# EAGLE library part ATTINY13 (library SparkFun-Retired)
ATTINY13 Retired
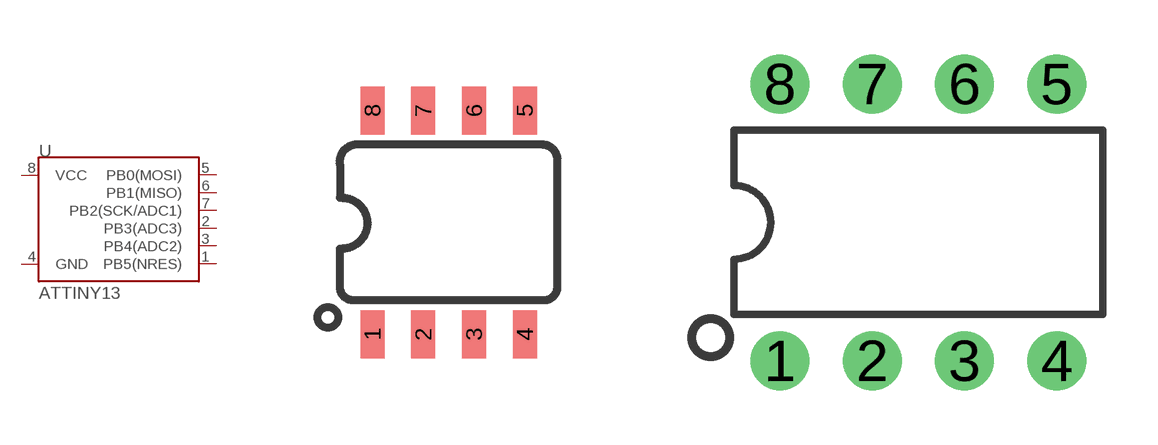
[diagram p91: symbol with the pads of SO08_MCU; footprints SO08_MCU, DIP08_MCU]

Designator prefix -

## ATTINY13SOIC  [SO08_MCU]
1  PB5(NRES)
2  PB3(ADC3)
3  PB4(ADC2)
4  GND
5  PB0(MOSI)
6  PB1(MISO)
7  PB2(SCK/ADC1)
8  VCC

## ATTINY13DIP  [DIP08_MCU]
Pads as for SO08_MCU

## Footprint SO08_MCU (pad centres in mm)
SOIC, 0.15 inch width
smd 0.6 x 1.2: 1 -1.905,-2.8; 2 -0.635,-2.8; 3 0.635,-2.8; 4 1.905,-2.8; 5 1.905,2.8; 6 0.635,2.8; 7 -0.635,2.8; 8 -1.905,2.8

## Footprint DIP08_MCU (pad centres in mm)
Dual In Line Package
drill 0.813 pad 1.626: 1 -3.81,-3.81; 2 -1.27,-3.81; 3 1.27,-3.81; 4 3.81,-3.81; 5 3.81,3.81; 6 1.27,3.81; 7 -1.27,3.81; 8 -3.81,3.81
